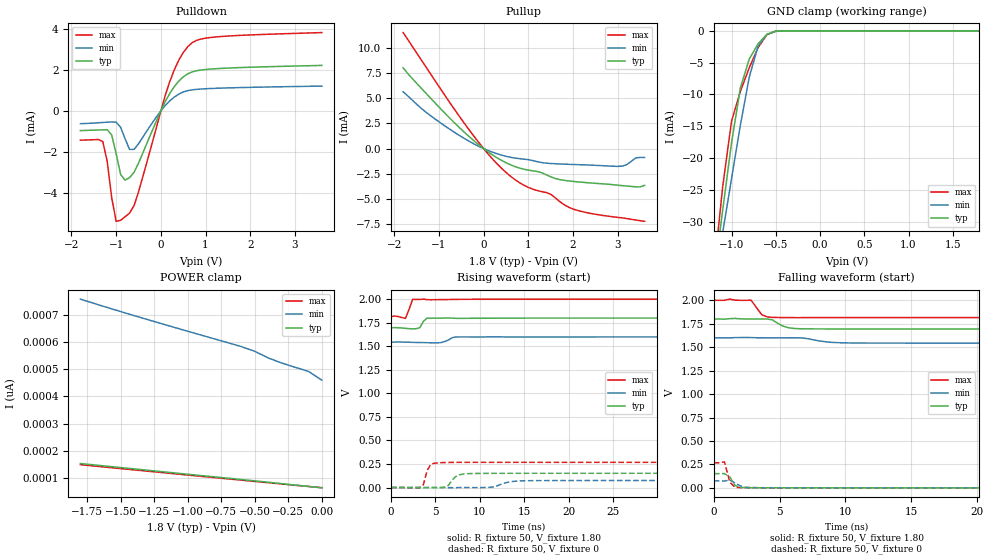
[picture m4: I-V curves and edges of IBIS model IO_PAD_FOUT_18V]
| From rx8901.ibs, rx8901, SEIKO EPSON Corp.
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[Model]   IO_PAD_FOUT_18V
Model_type 3-state
Enable Active-High
Polarity Non-Inverting
Vmeas=0.90
C_comp   2.5p   2.0p   3.0p
[Temperature Range] 25   105   -40
[Voltage Range]   1.80   1.60   2.00
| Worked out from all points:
|   slope of the pulldown table from 0 to 0.27 V, typ, clamps not added: 249 ohm
|   slope of the pullup table from 0 to 0.27 V, typ, clamps not added: 325 ohm
|   GND clamp passes 1 mA (typ) near -0.63 V on its own axis
|   falling waveform, R_fixture 50, V_fixture 1.80: 20-80 % time 889ps typ, 1.5ns min, 580ps max; typ from 1.8 V to 1.7 V
|   falling waveform, R_fixture 50, V_fixture 0: 20-80 % time 437ps typ, 626ps min, 345ps max; typ from 0.151 V to 0 V
|   rising waveform, R_fixture 50, V_fixture 1.80: 20-80 % time 463ps typ, 668ps min, 438ps max; typ from 1.7 V to 1.8 V
|   rising waveform, R_fixture 50, V_fixture 0: 20-80 % time 877ps typ, 1.49ns min, 570ps max; typ from 0 V to 0.151 V
[Pullup]
-1.8V     8.019mA    5.642mA    11.52mA
-1.3V     5.546mA    3.649mA    8.173mA
-500mV    1.91mA     1.186mA    2.939mA
100mV     -328.1uA   -188.8uA   -533.3uA
600mV     -1.606mA   -863uA     -2.738mA
1V        -2.14mA    -1.1mA     -3.857mA
1.5V      -2.802mA   -1.483mA   -4.534mA
1.8V      -3.153mA   -1.545mA   -5.569mA
2V        -3.258mA   -1.579mA   -6.004mA
3.1V      -3.677mA   -1.74mA    -6.882mA
3.4V      -3.796mA   -930.1uA   -7.094mA
3.6V      -3.649mA   -879uA     -7.222mA
[Pulldown]
-1.8V     -961.6uA   -625.3uA   -1.43mA
-1.3V     -922.8uA   -565.9uA   -1.492mA
-1.2V     -918.1uA   -551.9uA   -2.462mA
-1.1V     -1.178mA   -539uA     -4.238mA
-1V       -2.093mA   -553.4uA   -5.388mA
-900mV    -3.101mA   -802uA     -5.336mA
-700mV    -3.256mA   -1.879mA   -4.987mA
-600mV    -2.995mA   -1.879mA   -4.62mA
200mV     855.8uA    491.6uA    1.436mA
600mV     1.806mA    987.6uA    3.13mA
1.2V      2.053mA    1.099mA    3.601mA
3.6V      2.219mA    1.21mA     3.821mA
[GND Clamp]
-1.8V     -104.1mA   -93.3mA    -119.3mA
-1.2V     -38.9mA    -40.17mA   -37.89mA
-1.1V     -28.19mA   -31.69mA   -24.51mA
-1V       -17.59mA   -23.23mA   -14.19mA
-900mV    -8.967mA   -14.81mA   -9.505mA
-800mV    -4.445mA   -7.286mA   -5.815mA
-700mV    -2.032mA   -2.404mA   -2.638mA
-600mV    -545.5uA   -567.7uA   -606uA
-500mV    -57.02uA   -91.22uA   -35.65uA
-400mV    -3.189uA   -10.16uA   -752.6nA
1.8V      63.17pA    507.5pA    55.43pA
[POWER Clamp]
-1.8V     152.8pA    758.3pA    148.4pA
-1.3V     128.1pA    683.1pA    124.6pA
-600mV    93.83pA    583.5pA    91.48pA
-500mV    88.97pA    566.1pA    86.82pA
-400mV    83.98pA    541.8pA    82.2pA
-300mV    78.77pA    523pA      77.42pA
-100mV    68.42pA    492.2pA    68.29pA
0V        63.17pA    460pA      64.02pA
[Falling Waveform]
R_fixture=50
V_fixture=1.80
V_fixture_min=1.60
V_fixture_max=2.00
0s        1.8V       1.6V       2V
1.212ns   1.804V     1.6V       2.013V
2.828ns   1.8V       1.603V     2.001V
3.636ns   1.8V       1.6V       1.848V
4.444ns   1.792V     1.6V       1.818V
5.657ns   1.708V     1.6V       1.816V
6.869ns   1.696V     1.596V     1.815V
8.889ns   1.695V     1.552V     1.816V
10.51ns   1.694V     1.545V     1.816V
40ns      1.695V     1.544V     1.816V
[Falling Waveform]
R_fixture=50
V_fixture=0
V_fixture_min=0
V_fixture_max=0
0s        151.3mV    74.47mV    268mV
404ps     151.2mV    74.48mV    267.8mV
808.1ps   152.6mV    73.14mV    276.9mV
1.212ns   115.9mV    82.86mV    61.55mV
1.616ns   25.04mV    53.5mV     6.628mV
2.02ns    6.019mV    19.61mV    2.609mV
2.424ns   2.311mV    5.848mV    1.568mV
3.232ns   774.3uV    1.434mV    2.428mV
4.444ns   1.627mV    536.6uV    461.2uV
40ns      12.96uV    14.09uV    10.02uV
[Rising Waveform]
R_fixture=50
V_fixture=1.80
V_fixture_min=1.60
V_fixture_max=2.00
0s        1.695V     1.544V     1.816V
404ps     1.699V     1.545V     1.822V
1.616ns   1.691V     1.545V     1.797V
2.424ns   1.685V     1.542V     1.998V
3.232ns   1.698V     1.54V      1.998V
3.636ns   1.765V     1.54V      2.001V
4.04ns    1.799V     1.539V     1.996V
5.657ns   1.799V     1.541V     1.996V
7.273ns   1.797V     1.599V     1.998V
40ns      1.8V       1.6V       2V
[Rising Waveform]
R_fixture=50
V_fixture=0
V_fixture_min=0
V_fixture_max=0
0s        1.402nV    3.705nV    1.294nV
3.232ns   -568.6uV   26.95uV    -1.074mV
3.636ns   -2.395mV   25.37uV    30.26mV
4.04ns    -1.016mV   23.63uV    175.7mV
4.444ns   -148.5uV   25.73uV    243.3mV
5.253ns   -894.4uV   22.47uV    262.3mV
6.061ns   5.179mV    -286.5uV   265.7mV
8.485ns   146.7mV    -187.1uV   267.7mV
14.95ns   151.2mV    71.82mV    267.9mV
40ns      151.2mV    74.46mV    268mV
[Ramp]
R_load=50
dV/dt_r   9.074E-2/8.429E-10   4.468E-2/1.482E-9   1.608E-1/4.766E-10
dV/dt_f   6.318E-2/8.288E-10   3.371E-2/1.481E-9   1.106E-1/4.854E-10
|[End   IO_PAD_FOUT_18V
